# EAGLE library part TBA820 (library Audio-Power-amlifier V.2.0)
http://www.datasheetcatalog.com/datasheets_pdf/T/B/A/8/TBA820.shtml
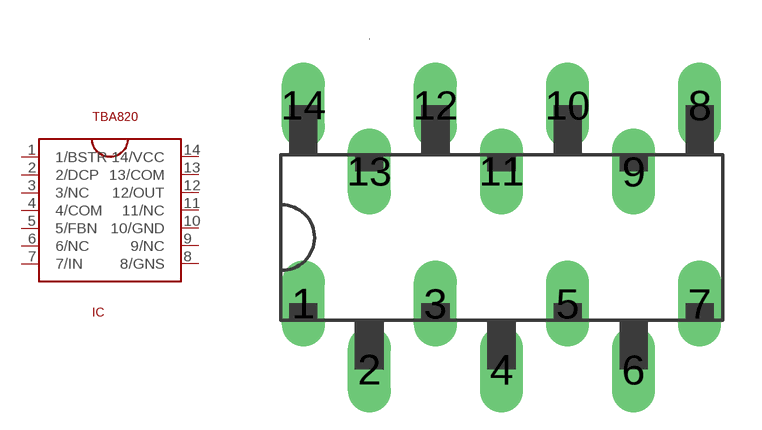
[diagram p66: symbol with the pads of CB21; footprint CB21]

Designator prefix IC

## TBA820  [CB21]
1  1/BSTR
2  2/DCP
3  3/NC  nc
4  4/COM
5  5/FBN
6  6/NC  nc
7  7/IN  in
8  8/GNS  pwr
9  9/NC  nc
10  10/GND  pwr
11  11/NC  nc
12  12/OUT  out
13  13/COM
14  14/VCC  pwr

## Footprint CB21 (pad centres in mm)
drill 1.1 long: 1 -7.62,-2.54; 2 -5.08,-5.08; 3 -2.54,-2.54; 4 0,-5.08; 5 2.54,-2.54; 6 5.08,-5.08; 7 7.62,-2.54; 8 7.62,5.08; 9 5.08,2.54; 10 2.54,5.08; 11 0,2.54; 12 -2.54,5.08; 13 -5.08,2.54; 14 -7.62,5.08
